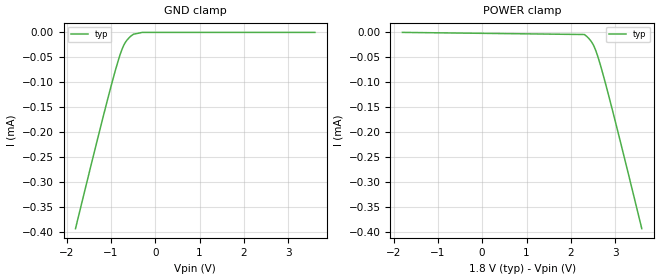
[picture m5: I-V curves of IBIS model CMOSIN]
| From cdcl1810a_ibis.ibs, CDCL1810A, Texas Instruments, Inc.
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|   Model CMOSIN
[Model]   CMOSIN
Model_type   Input
Vinl   = 6.00000e-001
Vinh   = 1.20000e+000
|   typ   min   max
C_comp   1.00000e-013   1.00000e-013   1.00000e-013
[Temperature Range]   2.70000e+001   NA   NA
|   |   typ   min   max
[Voltage Range]   1.80000e+000   NA   NA
[POWER Clamp Reference]   1.80000e+000   NA   NA
[GND Clamp Reference]   0.00000e+000   NA   NA
[GND Clamp]
| Voltage   I(typ)   I(min)   I(max)
-1.8V     -392.5uA   NA         NA
-1.235V   -189.4uA   NA         NA
-1.03V    -118.5uA   NA         NA
-895mV    -74.24uA   NA         NA
-805mV    -47.44uA   NA         NA
-720mV    -27.34uA   NA         NA
-640mV    -15.49uA   NA         NA
-555mV    -7.705uA   NA         NA
-495mV    -3.72uA    NA         NA
-295mV    2.212nA    NA         NA
3.6V      31.24pA    NA         NA
[POWER Clamp]
| Voltage   I(typ)   I(min)   I(max)
-1.8V     28.54pA    NA         NA
2.305V    -4.241uA   NA         NA
2.36V     -8.129uA   NA         NA
2.445V    -16.35uA   NA         NA
2.525V    -28.36uA   NA         NA
2.595V    -44.57uA   NA         NA
2.69V     -72.49uA   NA         NA
2.835V    -120.1uA   NA         NA
3.02V     -184.1uA   NA         NA
3.6V      -392.5uA   NA         NA
